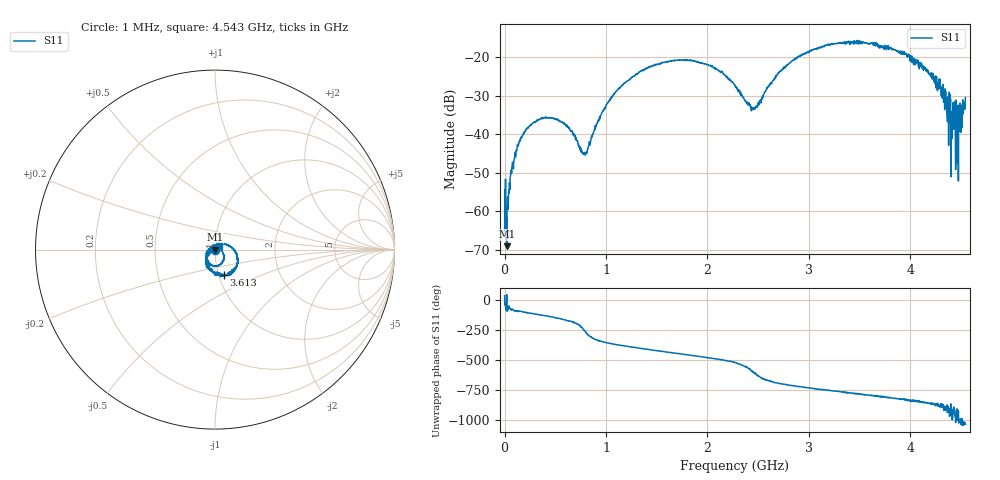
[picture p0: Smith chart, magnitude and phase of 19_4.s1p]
# HZ S RI R 50
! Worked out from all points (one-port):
!   1515 points, 1 MHz to 4.543 GHz, reference 50 ohm
!   lowest |S11| = -69.0 dB at 22 MHz (marker M1), VSWR 1.00, Z = 50 + j0.0263 ohm
!   |S11| at or under -10 dB: start of sweep to end of sweep
!   S11 on the Smith chart (normalised r, x): 1 MHz: 1.00, +0.00; 3.613 GHz: 1.06, -0.31; 4.543 GHz: 1.04, +0.05
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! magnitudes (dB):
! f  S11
! 1 MHz  -65.4
! 22 MHz  -69.0
! 61 MHz  -50.3
! 85 MHz  -47.3
! 139 MHz  -42.2
! 199 MHz  -39.4
! 385 MHz  -35.9
! 571 MHz  -37.0
! 793 MHz  -44.8
! 967 MHz  -34.1
! 1.138 GHz  -27.9
! 1.408 GHz  -22.8
! 1.705 GHz  -20.7
! 2.029 GHz  -22.1
! 2.272 GHz  -27.2
! 2.455 GHz  -33.5
! 2.692 GHz  -24.4
! 2.842 GHz  -20.7
! 3.181 GHz  -16.8
! 3.409 GHz  -16.6
! 3.613 GHz  -16.4
! 3.976 GHz  -19.8
! 4.291 GHz  -26.6
! 4.375 GHz  -33.8
! 4.393 GHz  -33.3
! 4.435 GHz  -31.7
! 4.459 GHz  -47.4
! 4.543 GHz  -30.4
